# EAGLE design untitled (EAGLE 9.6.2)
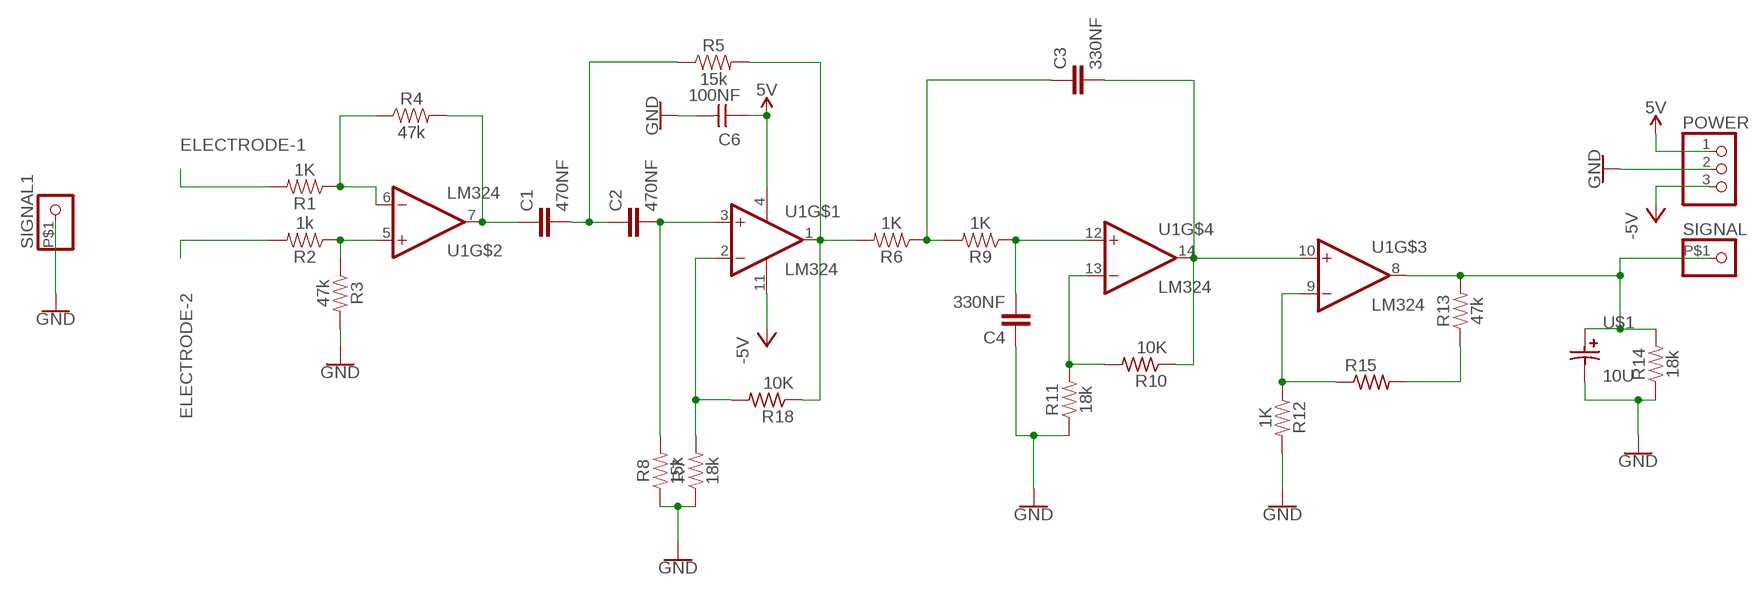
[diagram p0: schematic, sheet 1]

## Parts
C1  470NF  0.33UF/330NF-0805-50V-10%  [0805]
C2  470NF  0.33UF/330NF-0805-50V-10%  [0805]
C3  330NF  0.33UF/330NF-0805-50V-10%  [0805]
C4  330NF  0.33UF/330NF-0805-50V-10%  [0805]
C6  100NF  CAP_UNPOLARIZEDFAB  [C1206FAB]
POWER  PINHD-1X3  [1X03]
R1  1K  0.3OHM-0805-1/8W-1%  [0805]
R2  1k  0.3OHM-0805-1/8W-1%  [0805]
R3  47k  0.3OHM-0805-1/8W-1%  [0805]
R4  47k  0.3OHM-0805-1/8W-1%  [0805]
R5  15k  0.3OHM-0805-1/8W-1%  [0805]
R6  1K  0.3OHM-0805-1/8W-1%  [0805]
R7  18k  0.3OHM-0805-1/8W-1%  [0805]
R8  15k  0.3OHM-0805-1/8W-1%  [0805]
R9  1K  0.3OHM-0805-1/8W-1%  [0805]
R10  10K  R1206FAB  [R1206FAB]
R11  18k  0.3OHM-0805-1/8W-1%  [0805]
R12  1K  0.3OHM-0805-1/8W-1%  [0805]
R13  47k  0.3OHM-0805-1/8W-1%  [0805]
R14  18k  0.3OHM-0805-1/8W-1%  [0805]
R15  R1206FAB  [R1206FAB]
R18  10K  R1206FAB  [R1206FAB]
SIGNAL  PINHD-1X1-BIGPOGO  [1X1-BIGPOGO]
SIGNAL1  PINHD-1X1-BIGPOGO  [1X1-BIGPOGO]
U1  LM324  [SOIC127P600X175-14N]
U$1  10U  CAP_POLARIZED  [SMD-ELEC-CAP]

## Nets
5V: C6.1 POWER.1 U1.4(VCC+)
-5V: POWER.3 U1.11(VCC-)
ELECTRODE-1: R1.2
ELECTRODE-2: R2.2
GND: C4.1 C6.2 POWER.2 R3.2 R7.1 R8.1 R11.1 R12.2 R14.1 SIGNAL1.P$1 U$1.C
N$3: R2.1 R3.1 U1.5(NON-INVERTING_INPUT2)
N$4: R1.1 R4.1 U1.6(INVERTING_INPUT2)
N$5: C1.1 R4.2 U1.7(OUTPUT2)
N$6: C1.2 C2.1 R5.1
N$7: C2.2 R8.2 U1.3(NON-INVERTING_INPUT1)
N$8: C3.1 R6.1 R9.2
N$9: R5.2 R6.2 R18.1 U1.1(OUTPUT1)
N$10: R7.2 R18.2 U1.2(INVERTING_INPUT1)
N$11: C4.2 R9.1 U1.12(NON-INVERTING_INPUT4)
N$12: R12.1 R15.1 U1.9(INVERTING_INPUT3)
N$13: C3.2 R10.1 U1.10(NON-INVERTING_INPUT3) U1.14(OUTPUT4)
N$14: R13.1 R15.2
N$15: R10.2 R11.2 U1.13(INVERTING_INPUT4)
N$17: R13.2 R14.2 SIGNAL.P$1 U1.8(OUTPUT3) U$1.A

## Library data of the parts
C1-C4 = SparkFun-Capacitors:0.33UF/330NF: 0.33µF/330nF ceramic capacitors; PROD_ID: CAP-08469; VALUE: 0.33µF
C6 = fab:CAP_UNPOLARIZED
POWER = adafruit:PINHD-1X3: PIN HEADER
R1-R9 R11-R14 = SparkFun-Resistors:0.3OHM: 0.3Ω resistor; PROD_ID: RES-11622; VALUE: 0.3
R10 R15 R18 = fab:R: Resistor (US Symbol)
SIGNAL SIGNAL1 = adafruit:PINHD-1X1: Pin header 1x1 for 0.1" spacing
U1 = LM324:LM324: these devices consist of four independent high-gain frequency-compensated operational amplifiers that are designed sp...; DESCRIPTION: General Purpose Amplifier 4 Circuit 14-SOIC; MF: Texas Instruments; MP: LM324; PACKAGE: SOIC-14 Texas Instruments
U$1 = fab:CAP_POLARIZED

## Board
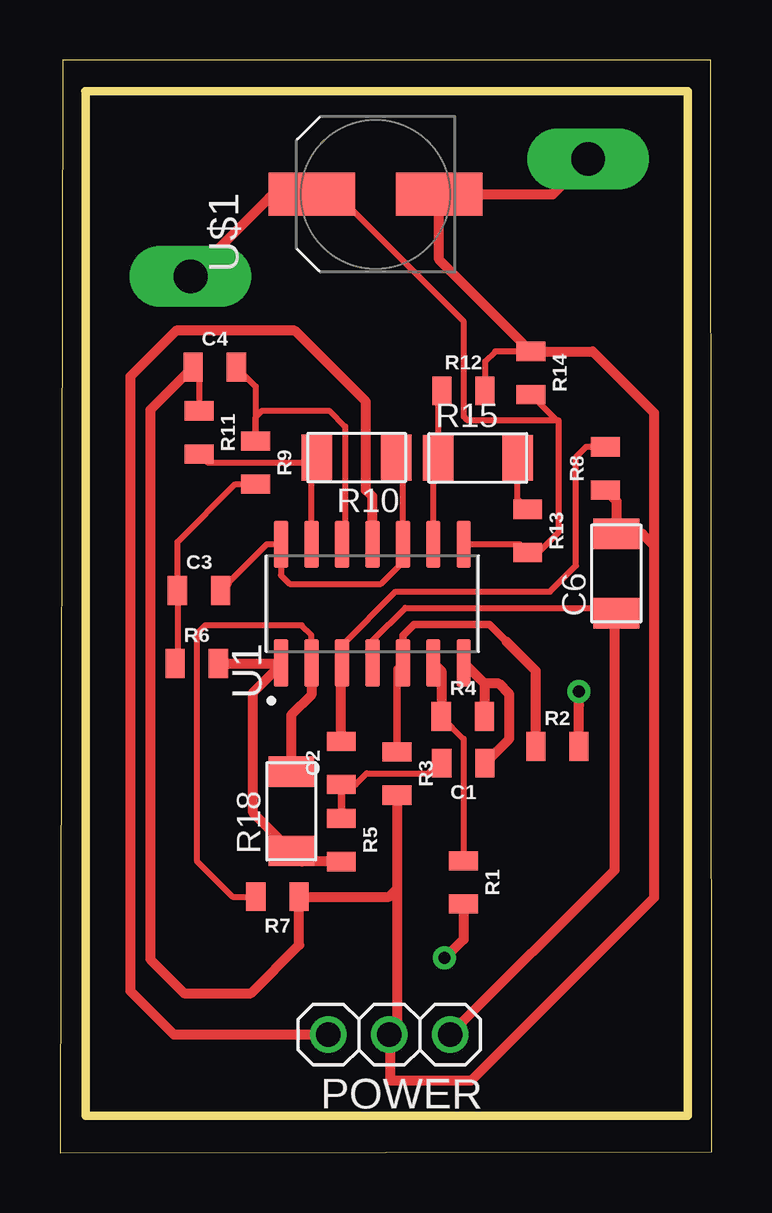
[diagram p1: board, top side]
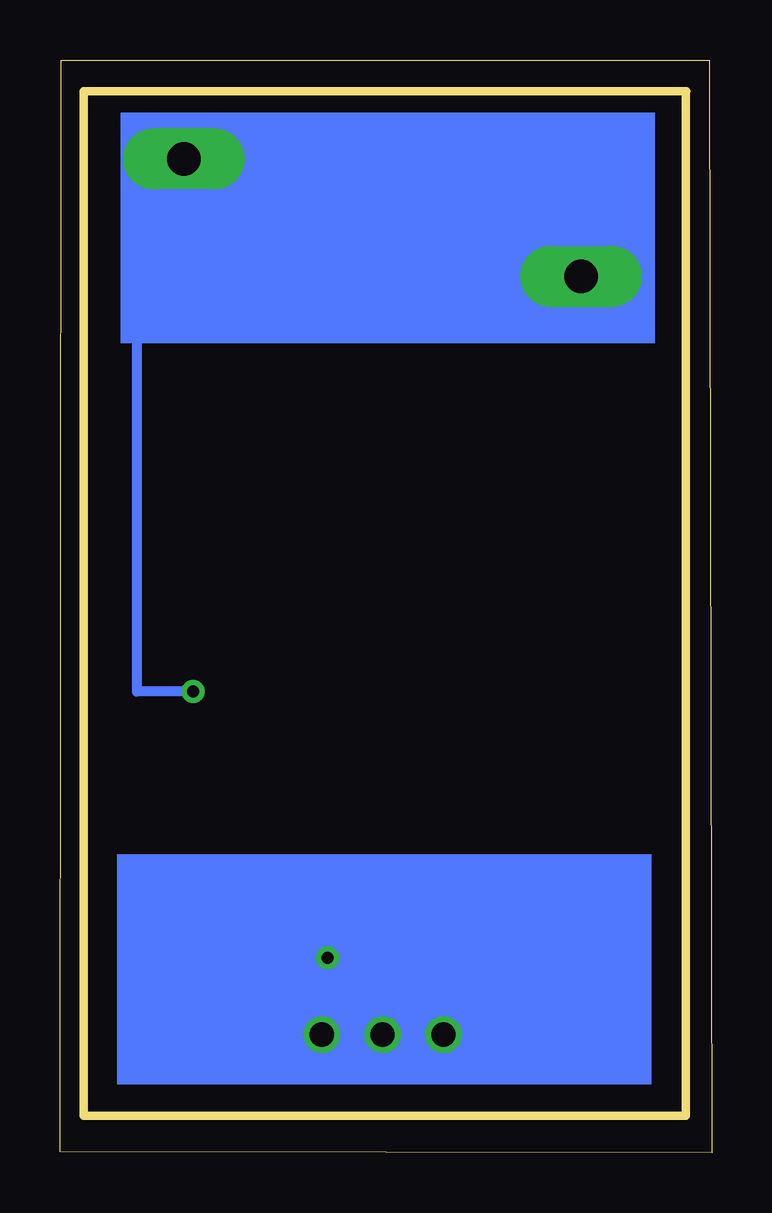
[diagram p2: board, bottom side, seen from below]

Size 27.18 x 45.54 mm. Coordinates in mm from the lower left corner, seen from the top.
Outline: 1.08,44.24 1.08,1.53 26.18,1.53 26.18,44.24 1.05,44.23
Outline: 0,0 27.18,0.03 27.13,45.53 0.11,45.54 0,0
Copper layers (1*16): Top 0.035mm / dielectric 1.5mm / Bottom 0.035mm
Design rules "default *": minimum track width 6mil, minimum drill 0.35mm, track to track 16mil, track to pad 16mil, pad to pad 16mil, via to via 16mil, smd to smd 16mil, copper to edge 40mil, drill to drill 6mil, minimum pad ring 10mil, minimum via ring 8mil, stop-mask expansion 10mil, vias tented up to drill 5mil, thermal gap 10mil

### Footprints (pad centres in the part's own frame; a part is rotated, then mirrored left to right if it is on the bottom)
0805 = smd 0.8 x 1.2: 1 -0.9,0; 2 0.9,0
C1206FAB = smd 1.27 x 1.905: 1 -1.651,0; 2 1.651,0
1X03 = drill 1.016: 1 -2.54,0; 2 0,0; 3 2.54,0
R1206FAB = smd 1.27 x 1.905: 1 -1.651,0; 2 1.651,0
1X1-BIGPOGO = drill 1.4 pad 2.54 long: P$1 0,0
SOIC127P600X175-14N = smd 1.97 x 0.6: 1 -2.475,3.81; 2 -2.475,2.54; 3 -2.475,1.27; 4 -2.475,0; 5 -2.475,-1.27; 6 -2.475,-2.54; 7 -2.475,-3.81; 8 2.475,-3.81; 9 2.475,-2.54; 10 2.475,-1.27; 11 2.475,0; 12 2.475,1.27; 13 2.475,2.54; 14 2.475,3.81
SMD-ELEC-CAP = smd 1.8 x 3.6: A 0,2.65; C 0,-2.65

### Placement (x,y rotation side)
C1  16.82,16.23 180 top
C2  11.73,16.24 90 top
C3  5.8,23.43 0 top
C4  6.45,32.74 0 top
C6  23.2,24.14 90 top
POWER  13.73,4.92 180 top
R1  16.83,11.26 270 top
R2  20.74,16.93 0 top
R3  14.05,15.8 270 top
R4  16.8,18.18 0 top
R5  11.73,13.03 270 top
R6  5.71,20.39 0 top
R7  9.07,10.67 180 top
R8  22.74,28.52 90 top
R9  8.16,28.76 270 top
R10  12.37,28.97 180 top
R11  5.8,30.02 270 top
R12  16.82,31.75 0 top
R13  19.5,25.92 270 top
R14  19.64,32.5 270 top
R15  17.42,28.96 0 top
R18  9.64,14.23 90 top
SIGNAL  5.45,36.52 180 top
SIGNAL1  22.02,41.42 0 top
U1  13.03,22.88 90 top
U$1  13.16,39.95 90 top

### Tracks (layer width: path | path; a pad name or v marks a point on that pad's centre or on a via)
5V
  Top 0.254: U1.4 13.03,21.34 14.4,22.71 22.98,22.71 23.13,22.56 C6.1
  Top 0.406: POWER.1 23.13,11.78 23.13,22.56
-5V
  Top 0.406: U1.11 13.03,27.35 12.76,27.62 12.76,31.3 9.8,34.26 4.84,34.26 2.93,32.35 2.93,6.73 4.75,4.92 POWER.3
ELECTRODE-1  (via drill 0.5 pad 0.95)
  Top 0.406: R1.2 16.83,8.88 16.06,8.12 v16.03,8.12
ELECTRODE-2  (via drill 0.5 pad 0.95)
  Top 0.406: R2.2 21.64,18.64 21.63,18.64 v21.63,19.22
  Bottom 0.406: v21.63,19.22 23.97,19.22 23.97,35.47 23.19,36.25
GND
  Top 0.254: C4.1 5.8,32.49 R11.1 | R14.1 18.15,33.4 17.72,32.97 R12.2
  Top 0.305: R3.2 14.02,14.86
  Top 0.406: R7.1 | R7.1 13.73,10.66 14.05,10.99 | R3.2 14.05,10.99 | 14.05,10.99 14.05,4.81 13.78,4.54 | POWER.2 13.78,4.97 13.78,4.54 | R8.1 23.2,27.15 C6.2 24.28,25.79 24.77,25.31 | 24.77,25.31 24.77,10.62 17.14,3 13.79,3 13.78,3.02 13.78,4.54 | 24.77,25.31 24.77,30.85 22.22,33.4 R14.1 15.8,37.23 U$1.C 20.54,39.95 SIGNAL1.P$1 | C4.1 3.76,30.95 3.76,8.06 5.17,6.65 7.97,6.65 9.97,8.65 R7.1
N$3
  Top 0.305: R3.1 14.05,20.16 U1.5 14.3,21.55 14.76,22.01 17.91,22.01 18.62,21.3 19.51,20.41
  Top 0.406: R2.1 19.84,20.08 18.62,21.3
N$4
  Top 0.203: 16.06,18.2 15.9,18.2
  Top 0.254: R4.1 16.83,17.25 R1.1
  Top 0.406: U1.6 15.9,20.08 15.9,18.2 R4.1
N$5
  Top 0.406: U1.7 17.7,19.55 | 17.7,19.55 R4.2 | C1.1 18.74,17.25 18.74,19.11 18.3,19.55 17.7,19.55
N$6
  Top 0.254: C2.1 12.32,15.34 12.79,15.81 15.35,15.81 15.74,16.2
  Top 0.305: C2.1 11.75,15.32 | 11.75,15.32 11.81,15.26 11.82,15.26 | 15.74,16.2 15.92,16.2 | R5.1 11.73,15.31 11.75,15.32
  Top 0.406: 15.92,16.2 C1.2 | C2.1
N$7
  Top 0.254: U1.3 11.76,21.14 13.99,23.38 20.43,23.38 21.51,24.46 21.51,28.98 21.95,29.42 R8.2
  Top 0.406: C2.2 11.73,20.38 U1.3
N$8
  Top 0.254: R6.1 4.9,20.48 C3.1 4.9,25.45 7.31,27.86 R9.2
  Top 0.305: C3.1
  Top 0.356: 4.9,23.81 C3.1
N$9
  Top 0.406: R5.2 10.09,12.13 R18.1 8.05,14.16 8.05,19.18 9.22,20.35 | 9.22,20.35 U1.1 | R6.2 9.17,20.39 9.22,20.35
N$10
  Top 0.254: U1.2 10.49,21.57 10.08,21.98 6.06,21.98 5.7,21.62 5.7,12.16 7.19,10.67 R7.2
  Top 0.406: U1.2 10.49,19.08 9.64,18.23 R18.2
N$11
  Top 0.254: U1.12 11.89,25.49 11.89,30.27 11.23,30.92 8.42,30.92 8.16,30.66 R9.1 8.16,31.93 C4.2
N$12
  Top 0.254: U1.9 15.57,28.75 R15.1 15.77,31.6 R12.1
N$13
  Top 0.254: C3.2 8.63,25.36 U1.14 9.22,24.06 9.58,23.7 13.38,23.7 14.3,24.62 U1.10 14.3,28.69 R10.1
  Top 0.356: C3.2 6.98,23.71
N$14
  Top 0.254: R13.1 19.07,27.24 R15.2
N$15
  Top 0.254: U1.13 10.49,28.74 R10.2 10.69,28.99 10.46,28.77 6.15,28.77 R11.2
N$17
  Top 0.254: U1.8 19.16,25.36 R13.2 19.96,25.02 20.8,25.86 20.8,30.52 20.71,30.52 | R14.2 20.71,30.52 | 20.71,30.52 16.99,30.52 16.84,30.68 16.84,34.64 | 16.84,34.64 16.84,34.65 | 16.84,34.64 11.67,39.81 10.59,39.81
  Top 0.406: SIGNAL.P$1 8.73,39.81 10.59,39.81 11.07,39.81 10.93,39.95 U$1.A
(copper drawn outside any net)
  shapes: Bottom area x2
